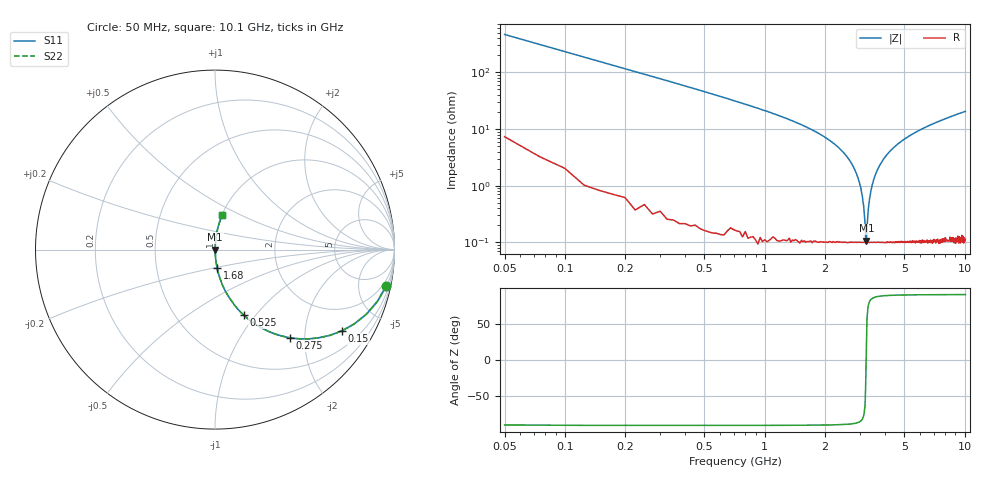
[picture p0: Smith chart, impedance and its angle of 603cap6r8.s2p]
! AVX Thin Film Operation		Date: November 2004
! Description: Accu-P® Series, Thin Film, SMD, RF Capacitor
! Part Number: 06035J6R8BBT
! 50 MHz  -  10.05 GHz
! Serial Measurements
# hz S db R 50
!	S11		S21		S12		S22
!	dB	Phase	dB	Phase	dB	Phase	dB	Phase
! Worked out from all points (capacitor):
!   400 points, 50 MHz to 10.1 GHz, reference 50 ohm
!   read as one part in series: C = 6.8 pF near 100 MHz
!   lowest |Z| = 107 mohm at 3.23 GHz (marker M1)
!   series resonance near 3.22 GHz, so ESL is about 360 pH
!   S11 on the Smith chart (normalised r, x): 50 MHz: 1.15, -9.37; 150 MHz: 1.02, -3.12; 275 MHz: 1.01, -1.69; 525 MHz: 1.00, -0.87; 1.68 GHz: 1.00, -0.20; 10.1 GHz: 1.00, +0.41
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5e7  -0.22 -12.0  -13.60 77.1  -13.60 77.1  -0.22 -12.0
1e8  -0.76 -23.1  -8.13 66.4  -8.13 66.4  -0.76 -23.1
1.5e8  -1.52 -32.6  -5.37 57.1  -5.37 57.1  -1.52 -32.6
2.75e8  -3.82 -49.7  -2.36 40.1  -2.36 40.1  -3.82 -49.7
5.25e8  -8.01 -66.4  -0.76 23.4  -0.76 23.4  -8.01 -66.4
1.68e9  -19.90 -83.6  -0.05 5.8  -0.05 5.8  -19.90 -83.6
1.73e9  -20.30 -83.9  -0.05 5.5  -0.05 5.5  -20.30 -83.9
2.43e9  -27.60 -86.2  -0.02 2.4  -0.02 2.4  -27.60 -86.2
2.88e9  -35.70 -85.6  -0.01 0.9  -0.01 0.9  -35.70 -85.6
3.08e9  -43.60 -81.0  -0.01 0.4  -0.01 0.4  -43.60 -81.0
3.13e9  -47.30 -76.4  -0.01 0.2  -0.01 0.2  -47.30 -76.4
3.18e9  -53.40 -62.1  -0.01 0.1  -0.01 0.1  -53.40 -62.1
3.2e9  -58.00 -37.1  -0.01 0.0  -0.01 0.0  -58.00 -37.1
3.23e9  -59.40 20.5  -0.01 -0.0  -0.01 -0.0  -59.40 20.5
3.3e9  -48.30 74.7  -0.01 -0.2  -0.01 -0.2  -48.30 74.7
3.4e9  -41.80 82.5  -0.01 -0.5  -0.01 -0.5  -41.80 82.5
3.6e9  -35.70 85.6  -0.01 -0.9  -0.01 -0.9  -35.70 85.6
3.95e9  -30.40 86.4  -0.01 -1.7  -0.01 -1.7  -30.40 86.4
5.08e9  -23.30 85.2  -0.03 -3.9  -0.03 -3.9  -23.30 85.2
6.75e9  -18.60 82.8  -0.07 -6.7  -0.07 -6.7  -18.60 82.8
8.43e9  -15.90 80.4  -0.12 -9.2  -0.12 -9.2  -15.90 80.4
1.01e10  -14.00 78.2  -0.19 -11.5  -0.19 -11.5  -14.00 78.2
